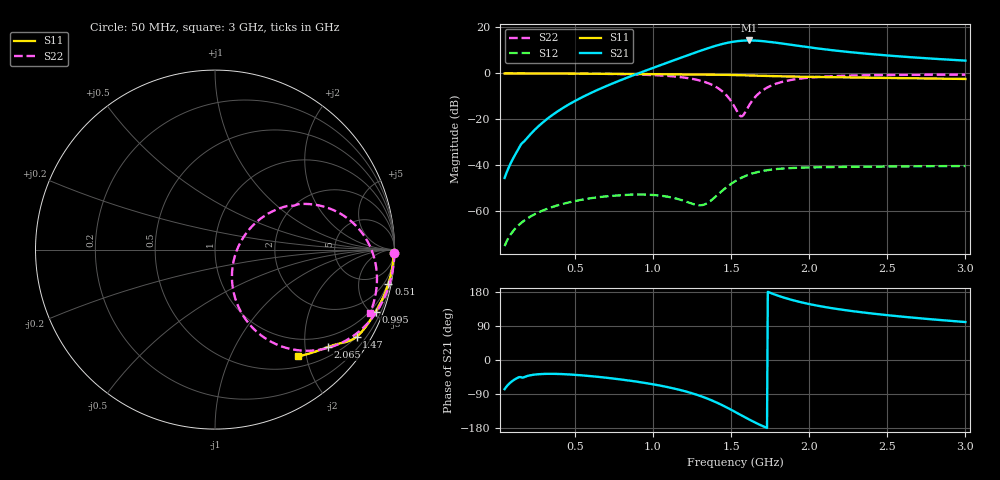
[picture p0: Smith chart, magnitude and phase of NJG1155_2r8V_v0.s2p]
! NJG1155UX2 S-parameter at VDD=2.8V
! Ver.0 2013-06-07
# hz S ma R 50
! freq  magS11  angS11  magS21  angS21  magS12  angS12  magS22  angS22
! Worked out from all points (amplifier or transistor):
!   591 points, 50 MHz to 3 GHz, reference 50 ohm
!   highest |S21| = 14.3 dB at 1.615 GHz (marker M1)
!   |S21| within 3 dB of that: 1.369 GHz to 2.001 GHz (632.2 MHz wide, 37.5 % of centre)
!   unconditionally stable (mu >= 1): 832.7 MHz to end of sweep
!   at 540 MHz: K = 0.45, MSG = 22.2 dB, |S12| = -54.9 dB
!   at 1.525 GHz: K = 3.49, MAG = 22.0 dB, |S12| = -46.9 dB
!   at 3 GHz: K = 1.77, MAG = 17.8 dB, |S12| = -40.3 dB
!   lowest NFmin = 0.40 dB at 725 MHz
!   S11 on the Smith chart (normalised r, x): 50 MHz: open; 510 MHz: 1, -10; 995 MHz: 0.61, -5.29; 1.47 GHz: 0.51, -3.47; 2.065 GHz: 0.72, -2.51; 3 GHz: 0.67, -1.86
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5e7  0.9956 -1.1  0.005342 -76.9  0.0001763 89.7  0.9999 -1.2
2.2e8  0.9935 -4.8  0.04932 -39.9  0.0007926 86.0  0.998 -5.3
5.1e8  0.9846 -11.1  0.2608 -39.4  0.00171 79.3  0.9876 -12.9
5.45e8  0.9831 -11.8  0.3007 -40.5  0.001802 78.5  0.9855 -13.9
7.95e8  0.971 -17.1  0.7139 -51.4  0.002253 72.4  0.9609 -22.0
9.95e8  0.9592 -21.1  1.292 -63.7  0.002286 69.0  0.917 -30.6
1.035e9  0.957 -22.0  1.449 -66.7  0.002226 68.9  0.903 -32.8
1.18e9  0.949 -24.9  2.189 -79.8  0.001777 73.8  0.8238 -42.1
1.285e9  0.9433 -27.2  2.935 -92.4  0.001373 97.5  0.7176 -51.2
1.375e9  0.9371 -29.2  3.715 -106.3  0.001769 134.6  0.5682 -60.4
1.47e9  0.9265 -31.5  4.548 -124.7  0.003341 146.4  0.3342 -67.8
1.525e9  0.9173 -32.9  4.918 -136.8  0.004511 143.2  0.1801 -58.4
1.565e9  0.9092 -33.8  5.089 -145.8  0.005361 138.8  0.1164 -17.6
1.615e9  0.8983 -34.8  5.168 -156.8  0.006327 132.2  0.2006 28.3
1.695e9  0.8812 -36.1  5.022 -173.0  0.007507 121.4  0.4094 33.1
1.805e9  0.8619 -37.6  4.539 169.0  0.008427 108.9  0.6208 23.6
1.9e9  0.849 -38.7  4.083 157.3  0.008816 101.0  0.7324 15.5
2.02e9  0.8357 -40.2  3.587 145.9  0.009069 93.7  0.8156 7.5
2.065e9  0.8312 -40.8  3.429 142.4  0.009131 91.6  0.8365 5.0
2.265e9  0.8126 -43.3  2.875 129.6  0.009319 84.7  0.8923 -3.8
2.51e9  0.7917 -46.3  2.425 117.9  0.009479 79.7  0.9204 -11.5
3e9  0.7544 -52.0  1.885 100.2  0.009699 74.9  0.9338 -22.3
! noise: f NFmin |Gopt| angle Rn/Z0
5e+07  1.252  0.9708  1.622  10.15
3.75e+08  0.4706  0.9133  8.157  1.152
7.05e+08  0.3977  0.8768  14.22  0.6859
1.03e+09  0.4121  0.853  20.03  0.5684
1.36e+09  0.4527  0.8264  25.35  0.5072
1.685e+09  0.5039  0.8024  31  0.4806
2.015e+09  0.5651  0.7783  36.72  0.4617
2.34e+09  0.6331  0.7549  42.32  0.4468
2.67e+09  0.7105  0.7317  47.93  0.4339
3e+09  0.7977  0.7091  53.43  0.4227
